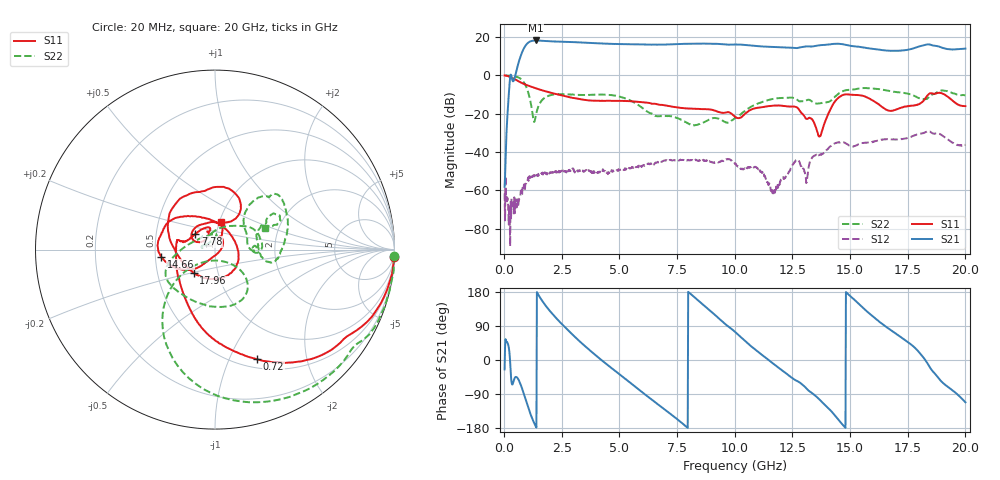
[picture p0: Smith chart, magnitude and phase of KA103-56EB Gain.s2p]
!Agilent Technologies,E8364B,MY43040668,A.07.50.67
!Agilent E8364B: A.07.50.67
!Date: Tuesday, November 27, 2018 09:53:37
!Correction: S11(Full 2 Port(1,2))
!S21(Full 2 Port(1,2))
!S12(Full 2 Port(1,2))
!S22(Full 2 Port(1,2))
!S2P File: Measurements: S11, S21, S12, S22:
# Hz S  dB  R 50
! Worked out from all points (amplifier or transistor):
!   1000 points, 20 MHz to 20 GHz, reference 50 ohm
!   highest |S21| = 18.3 dB at 1.36 GHz (marker M1)
!   |S21| within 3 dB of that: 910.2 MHz to 11.06 GHz (10.15 GHz wide, 170 % of centre)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
!   unconditionally stable (mu >= 1): 30.58 MHz to 42.32 MHz; 91.91 MHz to 118.9 MHz; 120.2 MHz to end of sweep
!   at 3.34 GHz: K = 18.33, MAG = 17.9 dB, |S12| = -49.9 dB
!   at 10.02 GHz: K = 16.05, MAG = 16.2 dB, |S12| = -46.4 dB
!   at 20 GHz: K = 5.70, MAG = 14.6 dB, |S12| = -36.2 dB
!   S11 on the Smith chart (normalised r, x): 20 MHz: 1, -46; 720 MHz: 0.60, -1.27; 7.78 GHz: 0.79, +0.14; 14.66 GHz: 0.54, -0.05; 17.96 GHz: 0.77, -0.21; 20 GHz: 1.02, +0.32
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2e7  -0.01 -2.5  -58.21 -24.8  -61.69 61.3  0.00 -2.2
7.2e8  -3.68 -69.0  10.28 -65.3  -60.59 -154.4  -1.77 -89.0
1.02e9  -5.23 -83.5  16.88 -121.2  -54.62 157.9  -8.02 -134.1
1.36e9  -6.66 -96.2  18.27 -173.8  -52.05 115.3  -21.79 -54.3
2.22e9  -9.61 -118.8  17.71 113.1  -50.63 56.0  -9.91 -64.4
3.36e9  -12.53 -154.9  17.21 44.5  -49.65 -2.7  -10.20 -114.8
4.68e9  -13.27 169.7  16.50 -22.4  -50.25 -51.9  -10.33 -154.9
5.7e9  -13.67 165.6  16.24 -71.2  -48.03 -87.5  -14.56 179.7
6.68e9  -15.12 164.9  16.07 -117.5  -45.34 -122.2  -21.30 112.3
7.78e9  -17.12 141.4  16.50 -169.8  -44.14 -158.2  -23.83 91.9
9.08e9  -18.20 103.4  16.53 122.3  -45.51 172.8  -22.25 169.3
1.002e10  -21.67 117.9  16.14 73.7  -46.38 141.7  -22.29 128.2
1.15e10  -15.99 145.4  14.96 -1.6  -56.40 128.4  -12.73 32.4
1.334e10  -22.76 55.5  15.15 -87.0  -43.31 -139.5  -13.53 -1.1
1.408e10  -19.46 -129.3  16.16 -128.7  -37.79 -174.3  -13.80 37.1
1.466e10  -10.35 -172.6  16.35 -169.6  -34.96 133.7  -8.34 49.6
1.562e10  -10.89 142.8  14.55 134.4  -35.21 96.4  -6.60 38.6
1.668e10  -18.43 41.7  12.93 82.6  -33.48 46.0  -8.13 7.4
1.796e10  -15.08 -131.9  15.01 22.8  -30.60 -8.7  -11.77 -7.8
1.836e10  -10.36 149.4  16.21 -9.4  -29.24 -37.9  -11.94 21.0
1.884e10  -9.11 86.2  15.15 -48.3  -30.30 -77.2  -8.33 31.8
2e10  -16.03 78.2  14.00 -111.5  -36.19 -117.1  -10.40 23.5
